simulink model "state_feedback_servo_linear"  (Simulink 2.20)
settings: Solver=ode1  StartTime=0.0  StopTime=999999  FixedStep=0.001  RelTol=1e-3  AbsTol=1e-6
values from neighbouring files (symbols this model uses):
  K = place(A,B,[lambda1,lambda2])    [design_state_feedback.m]    (also in design_state_feedback_obs.m)
  kc = 1/(C*inv(B*K-A)*B)    [design_state_feedback.m]    (also in design_state_feedback_obs.m)
libraries: winlib x3

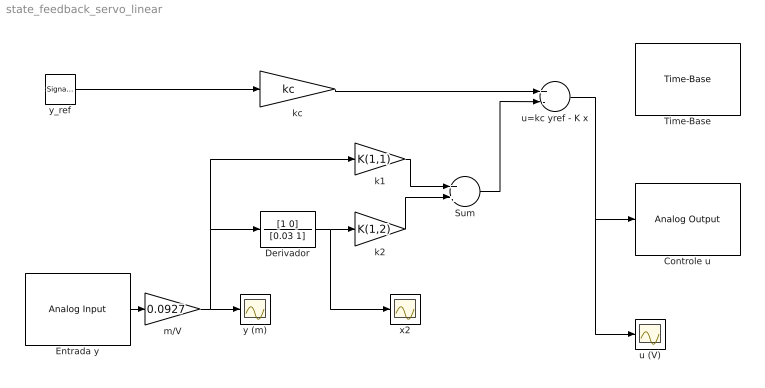
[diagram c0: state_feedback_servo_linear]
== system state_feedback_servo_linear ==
  Controle u : winlib/Quanser Consulting MultiQ Series/Analog Output  baseAddr=0x320  channels=[3]  initialOutputs=0  finalOutputs=0  sampleTime=str2num(get_param(bdroot, 'FixedStep'))
  Derivador : TransferFcn  Numerator=[1 0]  Denominator=[0.03 1]
  Entrada y : winlib/Quanser Consulting MultiQ Series/Analog Input  baseAddr=0x320  channels=[1]  sampleTime=str2num(get_param(bdroot, 'FixedStep'))
  Sum : Sum  Inputs=++
  Time-Base : winlib/Quanser Consulting MultiQ Series/Time-Base  baseAddr=0x320  irqLevel=9  clockSource=1
  k1 : Gain  Gain=K(1,1)
  k2 : Gain  Gain=K(1,2)
  kc : Gain  Gain=kc
  m/V : Gain  Gain=0.0927
  u (V) : Scope
  u=kc yref - K x : Sum  Inputs=+-
  x2 : Scope
  y (m) : Scope
  y_ref : SignalGenerator  WaveForm=square  Amplitude=0.05  Frequency=0.2  Units=Hertz
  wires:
  k2/1 -> Sum/2
  k1/1 -> Sum/1
  Sum/1 -> u=kc yref - K x/2
  u=kc yref - K x/1 -> Controle u/1, u (V)/1
  y_ref/1 -> kc/1
  kc/1 -> u=kc yref - K x/1
  Derivador/1 -> k2/1, x2/1
  Entrada y/1 -> m/V/1
  m/V/1 -> y (m)/1, Derivador/1, k1/1
